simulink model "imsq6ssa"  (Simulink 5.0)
settings: Solver=ode45  StartTime=0  StopTime=0.35  MaxStep=1e-5  RelTol=1e-3  AbsTol=1e-3
InitFcn:
  | ic=[ 0.8330    0.0019   -0.9472    0.0014   -0.9784    0.0078];
undefined symbols (not defined in the file or in its folder): sgn
libraries: simulink x1, mrlib x1

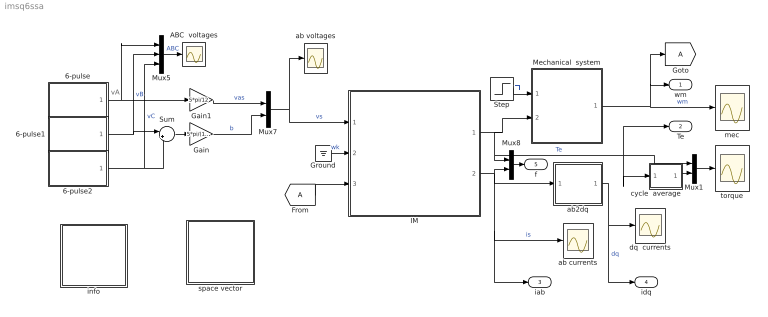
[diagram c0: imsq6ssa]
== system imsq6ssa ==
  note: vA
  6-pulse : Subsystem  mask{A=1, w=2*pi*50, p=1e-3}
      mask prompts: A "Amplitude"; w "Frequency [rad/s]"; p "Phase [rad]"
  6-pulse1 : Subsystem  mask{A=1.0, w=2*pi*50, p=-2*pi/3+1e-3}
      mask prompts: A "Amplitude"; w "Frequency [rad/s]"; p "Phase [rad]"
  6-pulse2 : Subsystem  mask{A=1.0, w=2*pi*50, p=2*pi/3+1e-3}
      mask prompts: A "Amplitude"; w "Frequency [rad/s]"; p "Phase [rad]"
  ABC  voltages : Scope
  Gain : Gain  Gain=5*pi/(12*sqrt(3))
  Gain1 : Gain  Gain=5*pi/12
  Ground : Ground
  IM : Subsystem  mask{Rs=0.01, Rr=0.02, Lsl=0.10, Lrl=0.10, Lm=4.5, wo=2*pi*60}
      mask prompts: Rs "Stator resistance [pu]"; Rr "Rotor resistance [pu]"; Lsl "Stator leakage inductance [pu]"; Lrl "Rotor leakage inductance [pu]"; Lm "Magnetizing inductance [pu]"; wo "Base frequency [rad/s]"
  Mechanical  system : Subsystem  mask{H=0.3, Bm=1e-5}
      mask prompts: H "Inertia constant [s]"; Bm "Torque-speed coefficient"
  Mux1 : Mux  Inputs=2
  Mux5 : Mux  Inputs=3
  Mux7 : Mux  Inputs=2
  Mux8 : Mux  Inputs=2
  Step : Step  Time=.05  SampleTime=0
  Sum : Sum  Inputs=|+-
  ab currents : Scope
  ab voltages : Scope
  ab2dq : Subsystem
  cycle  average : Subsystem
  dq  currents : Scope
  info : Subsystem
  mec : Scope
  space vector : Subsystem
  torque : Scope
  wm : Outport
  Te : Outport  Port=2
  iab : Outport  Port=3
  idq : Outport  Port=4
  f : Outport  Port=5
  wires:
  Sum/1 -> Gain/1
  6-pulse1/1(Out1) -> Sum/1, Mux5/2  "vB"
  6-pulse2/1(Out1) -> Sum/2, Mux5/3  "vC"
  6-pulse/1(Out1) -> Mux5/1, Gain1/1
  Mux5/1 -> ABC  voltages/1  "ABC"
  Gain/1 -> Mux7/2  "b"
  Gain1/1 -> Mux7/1  "vas"
  Mux7/1 -> ab voltages/1, IM/1(vs)  "vs"
  Ground/1 -> IM/2(wk)  "wk"
  Step/1 -> Mechanical  system/1(Tl)  "Tl"
  Mechanical  system/1(wm) -> mec/1, wm/1, [A]  "wm"
  IM/1(Te) -> Mechanical  system/2(Te), Mux8/1, Te/1, cycle  average/1(sig), Mux1/1  "Te"
  [A] -> IM/3(wm)
  ab2dq/1(dq) -> idq/1, dq  currents/1  "dq"
  Mux8/1 -> f/1
  IM/2(is) -> ab2dq/1(ab), ab currents/1, iab/1, Mux8/2  "is"
  Mux1/1 -> torque/1
  cycle  average/1(ave) -> Mux1/2

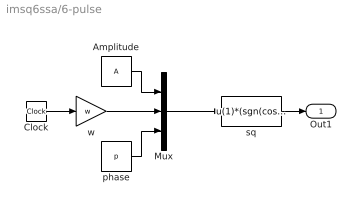
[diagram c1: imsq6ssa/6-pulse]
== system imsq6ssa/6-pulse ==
  Amplitude : Constant  Value=A
  Clock : Clock
  Mux : Mux  Inputs=3
  phase : Constant  Value=p
  sq : Fcn  Expr=u(1)*(sgn(cos(u(2)+u(3)))/2+sgn(cos(-3*(u(2)+u(3))))/6)
  w : Gain  Gain=w
  Out1 : Outport
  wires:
  Mux/1 -> sq/1
  sq/1 -> Out1/1
  Clock/1 -> w/1
  w/1 -> Mux/2
  phase/1 -> Mux/3
  Amplitude/1 -> Mux/1

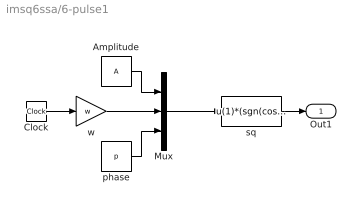
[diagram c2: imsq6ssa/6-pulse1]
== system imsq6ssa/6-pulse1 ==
  Amplitude : Constant  Value=A
  Clock : Clock
  Mux : Mux  Inputs=3
  phase : Constant  Value=p
  sq : Fcn  Expr=u(1)*(sgn(cos(u(2)+u(3)))/2+sgn(cos(-3*(u(2)+u(3))))/6)
  w : Gain  Gain=w
  Out1 : Outport
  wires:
  Amplitude/1 -> Mux/1
  phase/1 -> Mux/3
  w/1 -> Mux/2
  Clock/1 -> w/1
  sq/1 -> Out1/1
  Mux/1 -> sq/1

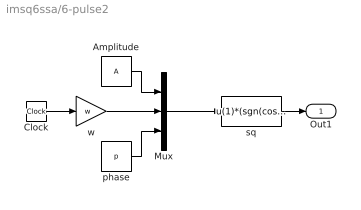
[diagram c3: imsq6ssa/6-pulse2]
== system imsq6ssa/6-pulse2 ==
  Amplitude : Constant  Value=A
  Clock : Clock
  Mux : Mux  Inputs=3
  phase : Constant  Value=p
  sq : Fcn  Expr=u(1)*(sgn(cos(u(2)+u(3)))/2+sgn(cos(-3*(u(2)+u(3))))/6)
  w : Gain  Gain=w
  Out1 : Outport
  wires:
  Mux/1 -> sq/1
  sq/1 -> Out1/1
  Clock/1 -> w/1
  w/1 -> Mux/2
  phase/1 -> Mux/3
  Amplitude/1 -> Mux/1

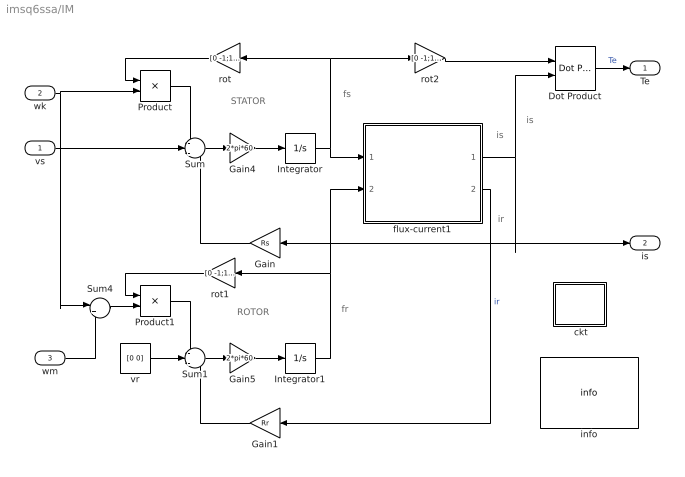
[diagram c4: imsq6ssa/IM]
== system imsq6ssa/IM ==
  note: ROTOR
  note: STATOR
  note: fs
  note: fr
  note: is
  note: is
  note: ir
  vs : Inport
  wk : Inport  Port=2
  wm : Inport  Port=3
  " ckt" : Subsystem
  Dot Product : simulink/Math Operations/Dot Product
  Gain : Gain  Orientation=left  Gain=Rs
  Gain1 : Gain  Orientation=left  Gain=Rr
  Gain4 : Gain  Gain=2*pi*60
  Gain5 : Gain  Gain=2*pi*60
  Integrator : Integrator  InitialCondition=[0 0]
  Integrator1 : Integrator  InitialCondition=[0 0]
  Product : Product
  Product1 : Product
  Sum : Sum  Inputs=-+-
  Sum1 : Sum  Inputs=-+-
  Sum4 : Sum  Inputs=|+-
  flux-current1 : Subsystem
  info : mrlib/IM/info
  rot : Gain  Orientation=left  Gain=[0 -1;1 0]  Multiplication=Matrix(K*u)
  rot1 : Gain  Orientation=left  Gain=[0 -1;1 0]  Multiplication=Matrix(K*u)
  rot2 : Gain  Gain=[0 -1;1 0]  Multiplication=Matrix(K*u)
  vr : Constant  Value=[0 0]
  Te : Outport
  is : Outport  Port=2
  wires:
  Gain/1 -> Sum/3
  vr/1 -> Sum1/2
  Gain1/1 -> Sum1/3
  flux-current1/2(ir) -> Gain1/1  "ir"
  Integrator/1 -> flux-current1/1(fs), rot/1, rot2/1
  Integrator1/1 -> flux-current1/2(fr), rot1/1
  Product1/1 -> Sum1/1
  rot1/1 -> Product1/1
  Product/1 -> Sum/1
  rot/1 -> Product/1
  rot2/1 -> Dot Product/1
  Sum4/1 -> Product1/2
  Sum/1 -> Gain4/1
  Gain4/1 -> Integrator/1
  Sum1/1 -> Gain5/1
  Gain5/1 -> Integrator1/1
  flux-current1/1(is) -> Gain/1, is/1, Dot Product/2
  Dot Product/1 -> Te/1  "Te"
  vs/1 -> Sum/2
  wk/1 -> Product/2, Sum4/1
  wm/1 -> Sum4/2

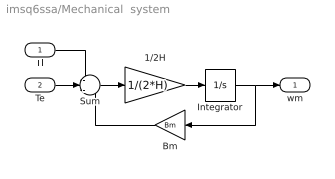
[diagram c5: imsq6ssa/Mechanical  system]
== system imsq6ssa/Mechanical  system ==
  Tl : Inport
  Te : Inport  Port=2
  1/2H : Gain  Gain=1/(2*H)
  Bm : Gain  Orientation=left  Gain=Bm
  Integrator : Integrator  InitialCondition=.82
  Sum : Sum  Inputs=-+-
  wm : Outport
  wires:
  Tl/1 -> Sum/1
  Te/1 -> Sum/2
  Integrator/1 -> wm/1, Bm/1
  Bm/1 -> Sum/3
  Sum/1 -> 1/2H/1
  1/2H/1 -> Integrator/1

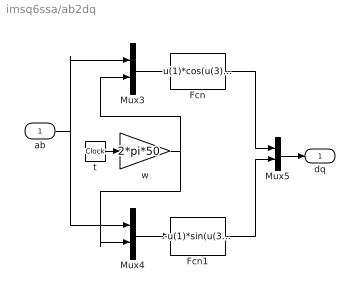
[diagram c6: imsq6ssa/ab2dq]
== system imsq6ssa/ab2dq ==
  ab : Inport
  Fcn : Fcn  Expr=u(1)*cos(u(3))+u(2)*sin(u(3))
  Fcn1 : Fcn  Expr=-u(1)*sin(u(3))+u(2)*cos(u(3))
  Mux3 : Mux  Inputs=2
  Mux4 : Mux  Inputs=2
  Mux5 : Mux  Inputs=2
  t : Clock
  w : Gain  Gain=2*pi*50
  dq : Outport
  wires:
  t/1 -> w/1
  Mux3/1 -> Fcn/1
  Mux4/1 -> Fcn1/1
  w/1 -> Mux3/2, Mux4/2
  ab/1 -> Mux3/1, Mux4/1
  Fcn1/1 -> Mux5/2
  Fcn/1 -> Mux5/1
  Mux5/1 -> dq/1

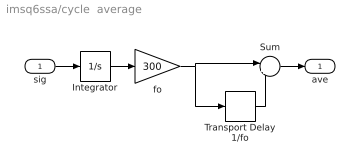
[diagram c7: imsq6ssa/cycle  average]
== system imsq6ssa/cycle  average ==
  sig : Inport
  Integrator : Integrator
  Sum : Sum  Inputs=|+-
  Transport Delay 1/fo : TransportDelay  DelayTime=1/300
  fo : Gain  Gain=300
  ave : Outport
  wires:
  Integrator/1 -> fo/1
  fo/1 -> Sum/1, Transport Delay 1/fo/1
  sig/1 -> Integrator/1
  Transport Delay 1/fo/1 -> Sum/2
  Sum/1 -> ave/1

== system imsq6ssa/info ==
  note: An induction motor under 6-pulse squarewave excitation
  note: The motor runs in a steady state at no load when a step load is suddenly applied.

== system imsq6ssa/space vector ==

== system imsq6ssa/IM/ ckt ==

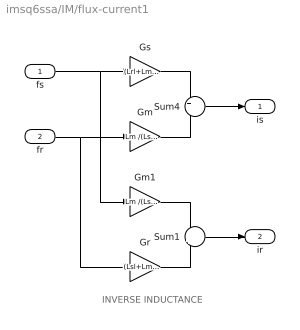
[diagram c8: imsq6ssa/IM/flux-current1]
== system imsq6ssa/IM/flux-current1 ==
  note: INVERSE INDUCTANCE
  fs : Inport
  fr : Inport  Port=2
  Gm : Gain  Gain=Lm /(Lsl*Lrl+Lsl*Lm+Lrl*Lm)
  Gm1 : Gain  Gain=Lm /(Lsl*Lrl+Lsl*Lm+Lrl*Lm)
  Gr : Gain  Gain=(Lsl+Lm )/(Lsl*Lrl+Lsl*Lm+Lrl*Lm)
  Gs : Gain  Gain=(Lrl+Lm) /(Lsl*Lrl+Lsl*Lm+Lrl*Lm)
  Sum1 : Sum  Inputs=-+
  Sum4 : Sum  Inputs=+-
  is : Outport
  ir : Outport  Port=2
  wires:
  fs/1 -> Gs/1, Gm1/1
  Gs/1 -> Sum4/1
  fr/1 -> Gm/1, Gr/1
  Gm/1 -> Sum4/2
  Sum4/1 -> is/1
  Gm1/1 -> Sum1/1
  Gr/1 -> Sum1/2
  Sum1/1 -> ir/1
